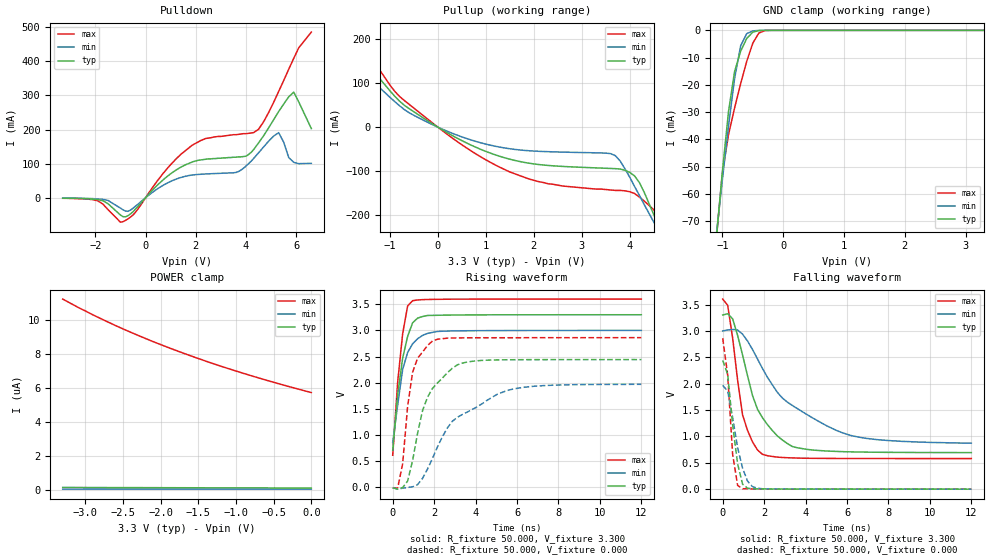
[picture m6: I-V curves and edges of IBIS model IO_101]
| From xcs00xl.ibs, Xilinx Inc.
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|   Model IO_101
[Model]   IO_101
Model_type   I/O
Polarity   Non-Inverting
Enable   Active-Low
Vinl =   0.800V
Vinh =   2.000V
Vmeas =   1.650V
Cref =  50.000pF
Rref =   1.000M
Vref =  0.000V
C_comp   5.300pF   3.500pF   6.800pF
[Temperature Range]   50.000   100.000   0.000
[Voltage Range]   3.300V   3.000V   3.600V
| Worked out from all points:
|   slope of the pulldown table from 0 to 0.495 V, typ, clamps not added: 12.8 ohm
|   slope of the pullup table from 0 to 0.495 V, typ, clamps not added: 16.3 ohm
|   GND clamp passes 1 mA (typ) near -0.52 V on its own axis
|   rising waveform, R_fixture 50.000, V_fixture 3.300: 20-80 % time 543ps typ, 571ps min, 408ps max; typ from 0.7 V to 3.3 V
|   rising waveform, R_fixture 50.000, V_fixture 0.000: 20-80 % time 1.12ns typ, 2.49ns min, 534ps max; typ from -0.012 V to 2.44 V
|   falling waveform, R_fixture 50.000, V_fixture 3.300: 20-80 % time 1.37ns typ, 3.04ns min, 714ps max; typ from 3.31 V to 0.694 V
|   falling waveform, R_fixture 50.000, V_fixture 0.000: 20-80 % time 421ps typ, 588ps min, 318ps max; typ from 2.44 V to 0.001 V
[Pulldown]
| voltage   I(typ)   I(min)   I(max)
-3.3V     -1.3mA     -1mA       -1.5mA
-1.9V     -5.4mA     -3.4mA     -9mA
-1V       -50.64mA   -30.43mA   -71.65mA
-700mV    -52.55mA   -39.74mA   -61.89mA
800mV     58.88mA    40.69mA    80.44mA
1.8V      103mA      66.09mA    151mA
3.6V      119mA      74.19mA    185mA
4V        122mA      93.03mA    188mA
4.5V      161mA      132mA      201mA
5.3V      253mA      191mA      312mA
5.9V      310mA      104mA      409mA
6.6V      203mA      101mA      486mA
[Pullup]
| voltage   I(typ)   I(min)   I(max)
-3.3V     56.96mA    11.83mA    218mA
-3.1V     77.62mA    14.78mA    321mA
-2.7V     251mA      38.7mA     345mA
-2.3V     242mA      180mA      297mA
-1.9V     198mA      157mA      238mA
-700mV    49.86mA    40.16mA    60.72mA
1.5V      -72.97mA   -49.19mA   -102mA
3.7V      -94.47mA   -64.95mA   -144mA
4.1V      -111mA     -135mA     -151mA
4.5V      -199mA     -216mA     -188mA
4.7V      -250mA     -255mA     -227mA
6.6V      -645mA     -572mA     -737mA
[GND_clamp]
| voltage   I(typ)   I(min)   I(max)
-3.3V     -539mA     -461mA     -635mA
-1.1V     -76.29mA   -74.81mA   -76.3mA
-1V       -51.66mA   -54.6mA    -52.25mA
-900mV    -29.77mA   -35.09mA   -38.23mA
-800mV    -15.1mA    -17.65mA   -28.49mA
-700mV    -7.645mA   -5.66mA    -19.53mA
-600mV    -2.968mA   -1.205mA   -11.34mA
-500mV    -649uA     -202uA     -4.68mA
-400mV    -83.34uA   -28.89uA   -976uA
-300mV    -8.303uA   -3.567uA   -95.2uA
3.3V      91.93nA    24.17nA    4.611uA
[POWER_clamp]
| voltage   I(typ)   I(min)   I(max)
-3.3V     126nA      27.82nA    11.23uA
-2.9V     121nA      27.69nA    10.3uA
-2.6V     117nA      27.29nA    9.671uA
-2.2V     113nA      27nA       8.903uA
-1.8V     109nA      25.98nA    8.207uA
-1.4V     104nA      25.35nA    7.571uA
-1V       101nA      24.85nA    6.988uA
-600mV    97.4nA     24.51nA    6.451uA
0V        91.95nA    23.79nA    5.718uA
[Ramp]
| variable   typ   min   max
dV/dt_r   1.465/1.101n   1.181/2.487n   1.717/0.501n
dV/dt_f   1.563/1.371n   1.276/3.036n   1.811/0.694n
R_load = 50.000
[Rising Waveform]
R_fixture = 50.000
V_fixture = 3.300
V_fixture_min = 3.000
V_fixture_max = 3.600
L_fixture = 0.000H
C_fixture = 0.000F
| time   V(typ)   V(min)   V(max)
0s        700mV      857mV      612mV
240ps     1.771V     1.571V     2.013V
480ps     2.468V     2.252V     2.934V
720ps     2.885V     2.577V     3.468V
960ps     3.144V     2.743V     3.568V
1.2ns     3.234V     2.84V      3.582V
1.44ns    3.265V     2.904V     3.588V
1.68ns    3.285V     2.942V     3.591V
2.16ns    3.289V     2.979V     3.594V
12ns      3.299V     2.999V     3.599V
[Rising Waveform]
R_fixture = 50.000
V_fixture = 0.000
V_fixture_min = 0.000
V_fixture_max = 0.000
L_fixture = 0.000H
C_fixture = 0.000F
| time   V(typ)   V(min)   V(max)
0s        -11.88mV   -7.26mV    -16.02mV
240ps     -35.24mV   -37.87mV   -15.1mV
480ps     -7.661mV   -18.35mV   449mV
720ps     118mV      -5.72mV    1.547V
960ps     508mV      7.221mV    2.198V
1.44ns    1.465V     168mV      2.585V
1.92ns    1.889V     550mV      2.796V
2.88ns    2.276V     1.262V     2.854V
5.52ns    2.438V     1.849V     2.859V
12ns      2.441V     1.968V     2.861V
[Falling Waveform]
R_fixture = 50.000
V_fixture = 3.300
V_fixture_min = 3.000
V_fixture_max = 3.600
L_fixture = 0.000H
C_fixture = 0.000F
| time   V(typ)   V(min)   V(max)
0s        3.305V     3.003V     3.608V
240ps     3.33V      3.022V     3.49V
480ps     3.232V     3.031V     2.867V
960ps     2.544V     2.941V     1.407V
1.44ns    1.776V     2.651V     896mV
1.92ns    1.356V     2.289V     661mV
2.64ns    1.01V      1.837V     608mV
3.36ns    810mV      1.589V     594mV
5.76ns    713mV      1.073V     583mV
12ns      694mV      873mV      581mV
[Falling Waveform]
R_fixture = 50.000
V_fixture = 0.000
V_fixture_min = 0.000
V_fixture_max = 0.000
L_fixture = 0.000H
C_fixture = 0.000F
| time   V(typ)   V(min)   V(max)
0s        2.445V     1.971V     2.864V
240ps     2.18V      1.86V      2.166V
480ps     1.22V      1.359V     659mV
720ps     481mV      787mV      70.33mV
960ps     94.77mV    398mV      8.852mV
1.2ns     18.16mV    152mV      7.106mV
1.44ns    7.853mV    47.06mV    4.281mV
1.68ns    5.485mV    17.85mV    3.408mV
1.92ns    6.263mV    7.829mV    2.964mV
12ns      502uV      665uV      338uV
